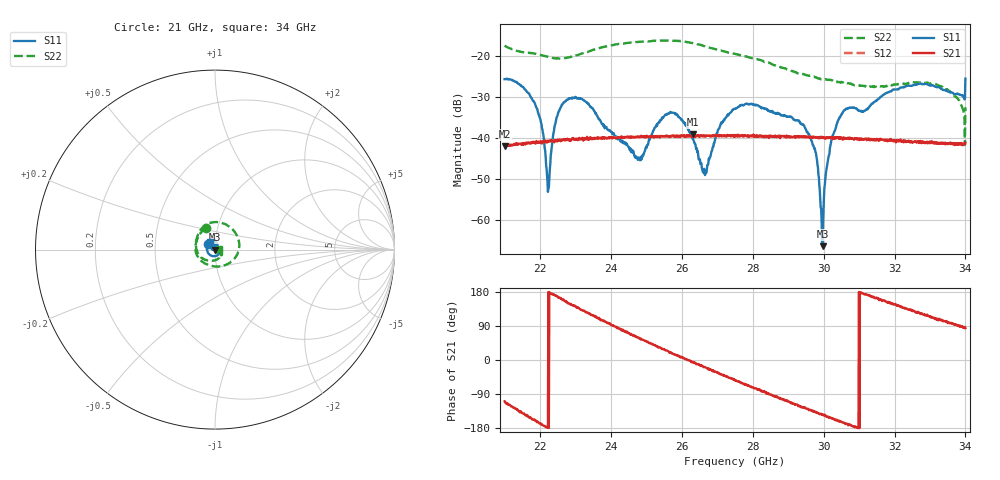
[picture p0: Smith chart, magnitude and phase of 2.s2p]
! 3/6/2025 3:18:09 PM
! C:\USERS\VECTORSTARUSER\DESKTOP\NEW FOLDER\2.S2P
! CHANNEL.1
! TR.MEASUREMENT
! CORRECTED.DATA
! RF.CORRECTION: FULL.TWO.PORT.CAL.PORT.1.2
! AVERAGING.OFF
! IF.BANDWIDTH: NO.IFBW
! SWEEPTYPE:  FREQ.SWEEP(Linear)
! Reference Plane Port Info
! PORT:  PORT1  PORT2
! DISTANCE:  0  m  0  m
! TIME:  0  s  0  s
! PHASE.OFFSET:  0 °  0 °
! LOSS:  0  dB  0  dB
! REF.LOSS:  0  dB  0  dB
! REF.FREQ:  0  Hz  0  Hz
! Power Info
! POWER:  -10  dBm  -10  dBm
! EFF.POWER:  -10  dBm  -10  dBm
! SOURCE.ATTEN:  0  dB  0  dB
! TEST.ATTEN:  0  dB  0  dB
# GHZ S RI R 50.0
! FREQ.GHZ  S11RE  S11IM  S21RE  S21IM  S12RE  S12IM  S22RE  S22IM
!; PortSelection: Port_12
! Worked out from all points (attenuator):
!   1001 points, 21 GHz to 34 GHz, reference 50 ohm
!   highest |S21| = -39.10 dB at 26.32 GHz (marker M1); lowest = -42.0 dB at 21.01 GHz (marker M2)
!   lowest |S11| = -66.4 dB at 29.97 GHz (marker M3), VSWR 1.00, Z = 50 - j0.0478 ohm
!   |S11| at or under -10 dB: start of sweep to end of sweep
!   |S22| runs from -41.7 to -16.2 dB; largest |S21 - S12| = 0.00069
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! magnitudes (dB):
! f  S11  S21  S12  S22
! 21 GHz  -25.7  -41.7  -42.0  -17.5
! 21.01 GHz  -25.7  -42.0  -41.7  -17.6
! 21.86 GHz  -31.7  -41.1  -41.0  -19.5
! 22.05 GHz  -37.5  -41.4  -40.9  -19.8
! 22.22 GHz  -53.1  -40.7  -40.7  -20.2
! 22.56 GHz  -32.9  -40.4  -40.6  -20.6
! 23.17 GHz  -30.4  -40.1  -40.1  -19.4
! 24.77 GHz  -45.0  -39.6  -39.7  -16.6
! 25.34 GHz  -36.2  -39.7  -39.5  -16.3
! 25.81 GHz  -33.9  -39.6  -39.5  -16.3
! 26.32 GHz  -40.2  -39.1  -39.5  -16.9
! 26.64 GHz  -48.5  -39.5  -39.6  -17.6
! 27.07 GHz  -37.3  -39.3  -39.4  -18.6
! 27.5 GHz  -32.9  -39.6  -39.6  -19.5
! 29.07 GHz  -34.8  -39.6  -39.6  -23.6
! 29.67 GHz  -40.9  -39.8  -39.7  -25.0
! 29.97 GHz  -66.4  -40.0  -39.9  -25.6
! 30.18 GHz  -42.4  -39.8  -39.8  -25.8
! 30.46 GHz  -35.0  -40.1  -40.0  -26.4
! 31.84 GHz  -28.8  -40.7  -40.5  -27.1
! 33.14 GHz  -27.5  -41.4  -41.0  -26.7
! 34 GHz  -25.5  -41.1  -41.1  -32.5
